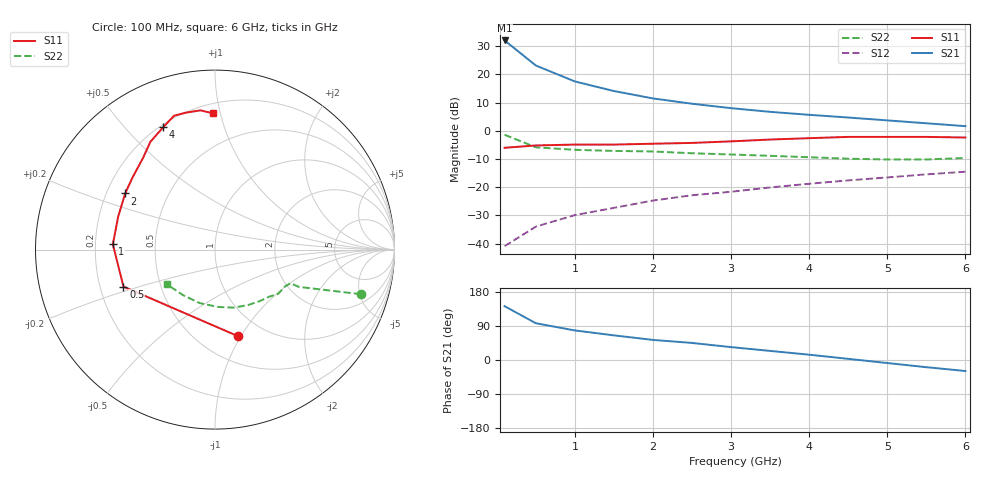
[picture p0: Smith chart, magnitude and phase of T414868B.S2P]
!AT-41486
!S-PARAMETERS at Vce=8V  Ic=25mA.  LAST UPDATED 07-21-92
# ghz s ma r 50
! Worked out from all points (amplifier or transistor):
!   13 points, 100 MHz to 6 GHz, reference 50 ohm
!   highest |S21| = 32.0 dB at 100 MHz (marker M1)
!   |S21| within 3 dB of that: start of sweep to 235 MHz
!   unconditionally stable (mu >= 1): 1.098 GHz to 3.146 GHz
!   at 1 GHz: K = 0.97, MSG = 23.7 dB, |S12| = -29.9 dB
!   at 3 GHz: K = 1.04, MAG = 13.5 dB, |S12| = -21.6 dB
!   at 6 GHz: K = 0.80, MSG = 8.1 dB, |S12| = -14.5 dB
!   S11 on the Smith chart (normalised r, x): 100 MHz: 0.76, -0.97; 500 MHz: 0.30, -0.18; 1 GHz: 0.27, +0.02; 2 GHz: 0.28, +0.27; 4 GHz: 0.21, +0.64; 6 GHz: 0.26, +0.95
0.1  0.5 -75.0  40.01 142.0  0.009 54.0  0.85 -17.0
0.5  0.55 -158.0  14.38 97.0  0.02 48.0  0.51 -24.0
1  0.57 177.0  7.5 78.0  0.032 61.0  0.46 -24.0
1.5  0.57 161.0  5.07 65.0  0.043 62.0  0.44 -28.0
2  0.59 148.0  3.75 53.0  0.058 59.0  0.43 -35.0
2.5  0.61 139.0  3.02 45.0  0.072 58.0  0.4 -41.0
3  0.65 128.0  2.52 34.0  0.083 57.0  0.38 -49.0
3.5  0.7 121.0  2.17 24.0  0.099 56.0  0.36 -59.0
4  0.74 113.0  1.92 14.0  0.115 52.0  0.34 -72.0
4.5  0.78 107.0  1.72 3.0  0.132 47.0  0.32 -87.0
5  0.78 102.0  1.53 -8.0  0.149 42.0  0.31 -106.0
5.5  0.78 96.0  1.36 -19.0  0.169 36.0  0.31 -125.0
6  0.76 91.0  1.21 -29.0  0.188 31.0  0.33 -144.0
